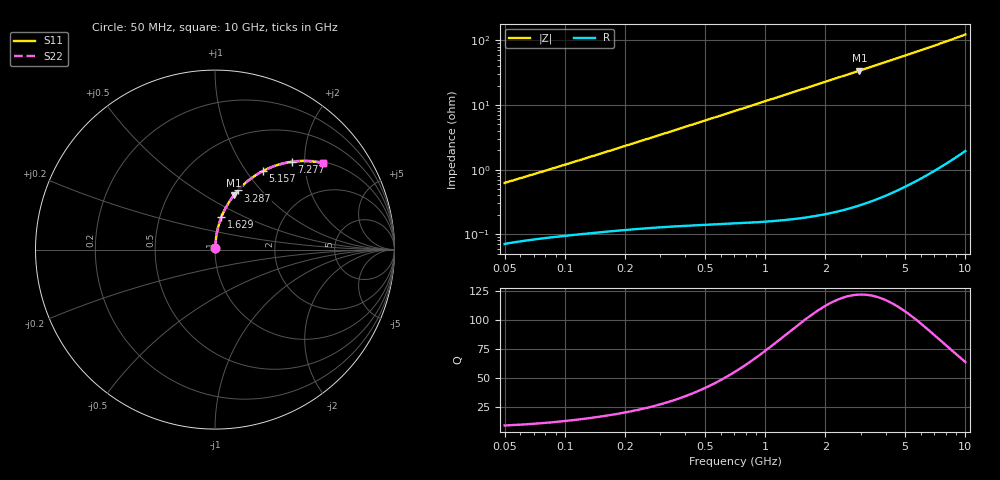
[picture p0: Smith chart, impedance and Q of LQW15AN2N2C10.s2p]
!Murata Part Number: LQW15AN2N2C10
!These Parameters are Measured in Series Mode Connection
!  o--[Z]--o
!Port1  Port2
!  o-------o
!Freq. Start=50[MHz] Stop=10[GHz], 401[Steps]
# Hz S RI R 50
!Freq.(Hz)	S 11(Real)	S 11(Imag)	S 21(Real)	S 21(Imag)	S 12(Real)	S 12(Imag)	S 22(Real)	S 22(Imag)
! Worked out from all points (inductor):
!   401 points, 50 MHz to 10 GHz, reference 50 ohm
!   read as one part in series: L = 1.93 nH near 51.34 MHz
!   highest Q = 122 at 2.956 GHz (marker M1), where L = 1.83 nH
!   S11 on the Smith chart (normalised r, x): 50 MHz: 1.00, +0.01; 1.629 GHz: 1.00, +0.37; 3.287 GHz: 1.01, +0.76; 5.157 GHz: 1.01, +1.20; 7.277 GHz: 1.02, +1.73; 10 GHz: 1.04, +2.47
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5e7  0.000744 0.00618  0.9993 -0.00618  0.9993 -0.00618  0.000744 0.00618
5.134228e7  0.000756 0.00633  0.9992 -0.00633  0.9992 -0.00633  0.000756 0.00633
6.780773e7  0.000884 0.0082  0.9991 -0.0082  0.9991 -0.0082  0.000884 0.0082
1.214486e8  0.00121 0.0143  0.9988 -0.0143  0.9988 -0.0143  0.00121 0.0143
2.949953e8  0.00242 0.0339  0.9976 -0.0339  0.9976 -0.0339  0.00242 0.0339
4.689809e8  0.00426 0.0535  0.9957 -0.0535  0.9957 -0.0535  0.00426 0.0535
7.071068e8  0.00795 0.0802  0.992 -0.0802  0.992 -0.0802  0.00795 0.0802
1.094763e9  0.017 0.123  0.983 -0.123  0.983 -0.123  0.017 0.123
1.335391e9  0.0244 0.1489  0.9756 -0.1489  0.9756 -0.1489  0.0244 0.1489
1.628911e9  0.0353 0.1796  0.9647 -0.1796  0.9647 -0.1796  0.0353 0.1796
1.717543e9  0.0389 0.1887  0.9611 -0.1887  0.9611 -0.1887  0.0389 0.1887
2.298604e9  0.0668 0.2455  0.9332 -0.2455  0.9332 -0.2455  0.0668 0.2455
2.956399e9  0.1056 0.3033  0.8944 -0.3033  0.8944 -0.3033  0.1056 0.3033
3.286879e9  0.1274 0.3294  0.8726 -0.3294  0.8726 -0.3294  0.1274 0.3294
3.703027e9  0.1566 0.3593  0.8434 -0.3593  0.8434 -0.3593  0.1566 0.3593
4.171863e9  0.1913 0.389  0.8087 -0.389  0.8087 -0.389  0.1913 0.389
5.156693e9  0.2675 0.438  0.7325 -0.438  0.7325 -0.438  0.2675 0.438
6.207365e9  0.3496 0.4716  0.6504 -0.4716  0.6504 -0.4716  0.3496 0.4716
7.276762e9  0.4297 0.4891  0.5703 -0.4891  0.5703 -0.4891  0.4297 0.4891
8.530394e9  0.5156 0.493  0.4844 -0.493  0.4844 -0.493  0.5156 0.493
9.738562e9  0.5887 0.4845  0.4113 -0.4845  0.4113 -0.4845  0.5887 0.4845
1e10  0.6033 0.4814  0.3967 -0.4814  0.3967 -0.4814  0.6033 0.4814
